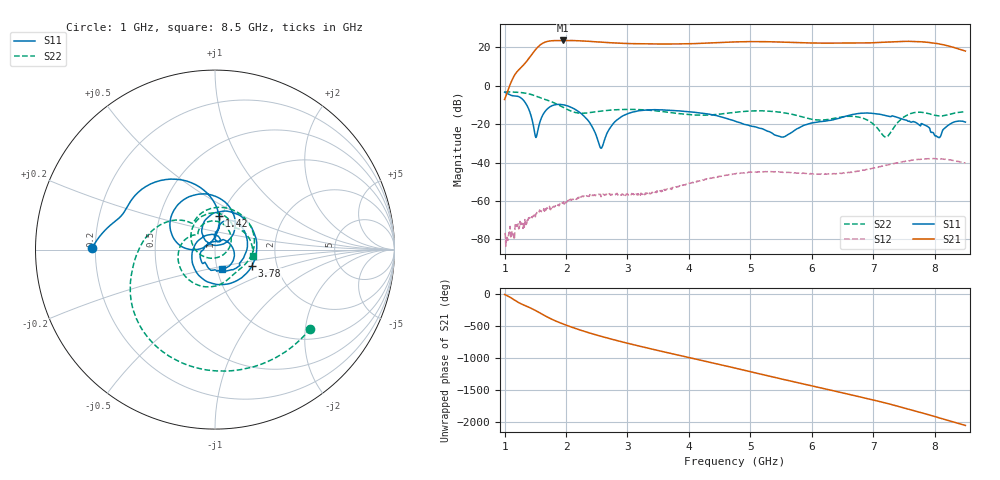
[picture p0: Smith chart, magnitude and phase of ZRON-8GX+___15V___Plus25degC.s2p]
!Mini-Circuits Laboratory
!S-Parameters
!Model:ZRON-8G+
!Run/Lot/Date Code:N/A
!Fixture/SN/Due: N/A
!Connection:PORT<1> - INPUT, PORT<2> - OUTPUT;
!Tested With: Network Analyzer E5071C
!Created: 11-30-2010 at 13:57:46
!S/N: Unit 1
#MHz S dB R 50
!Frequency  S11 dB  S11 DEG  S21 dB  S21 DEG  S12 dB  S12 DEG  S22 dB  S22 DEG
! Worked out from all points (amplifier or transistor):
!   751 points, 1 GHz to 8.5 GHz, reference 50 ohm
!   highest |S21| = 23.6 dB at 1.95 GHz (marker M1)
!   |S21| within 3 dB of that: 1.556 GHz to 8.239 GHz (6.683 GHz wide, 136 % of centre)
!   unconditionally stable (mu >= 1): start of sweep to end of sweep
!   at 2.25 GHz: K = 24.79, MAG = 23.7 dB, |S12| = -58.0 dB
!   at 4.75 GHz: K = 6.75, MAG = 23.1 dB, |S12| = -46.0 dB
!   at 8.5 GHz: K = 6.07, MAG = 18.4 dB, |S12| = -40.2 dB
!   S11 on the Smith chart (normalised r, x): 1 GHz: 0.19, +0.01; 1.42 GHz: 0.97, +0.38; 3.78 GHz: 1.49, -0.28; 8.5 GHz: 1.05, -0.23
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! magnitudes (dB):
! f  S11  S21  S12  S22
! 1 GHz  -3.3  -7.1  -76.8  -3.2
! 1.13 GHz  -5.2  3.6  -75.8  -3.2
! 1.28 GHz  -6.7  9.9  -72.0  -3.6
! 1.42 GHz  -14.5  15.4  -69.0  -4.4
! 1.51 GHz  -27.0  19.1  -66.7  -5.4
! 1.68 GHz  -12.5  23.0  -63.9  -7.3
! 1.95 GHz  -9.9  23.6  -61.1  -11.2
! 2.25 GHz  -14.6  23.4  -58.0  -14.3
! 2.57 GHz  -32.6  22.8  -57.8  -13.2
! 2.72 GHz  -21.8  22.5  -56.9  -12.7
! 2.9 GHz  -16.1  22.2  -57.0  -12.4
! 3.5 GHz  -12.5  21.8  -55.1  -13.2
! 3.78 GHz  -13.0  21.8  -52.9  -14.3
! 4.75 GHz  -18.5  22.9  -46.0  -13.8
! 5.52 GHz  -26.7  22.8  -45.0  -13.9
! 6 GHz  -19.4  22.3  -45.8  -17.5
! 6.77 GHz  -14.4  22.3  -44.4  -16.4
! 7.25 GHz  -15.9  22.9  -41.1  -25.8
! 7.6 GHz  -18.8  23.2  -39.0  -14.6
! 8.06 GHz  -26.9  21.9  -38.0  -15.7
! 8.26 GHz  -19.7  20.5  -38.6  -14.8
! 8.5 GHz  -18.9  18.1  -40.2  -13.5
